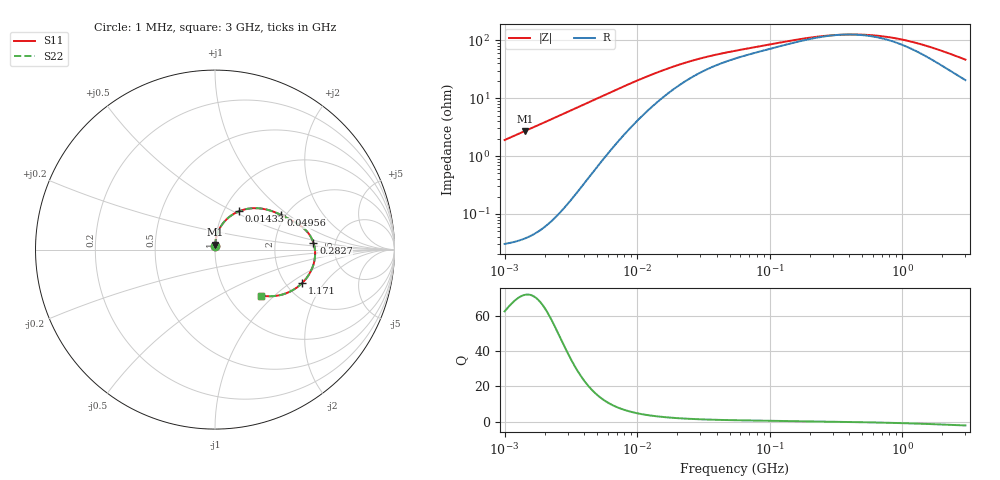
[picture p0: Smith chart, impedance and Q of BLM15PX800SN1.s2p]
! BLM15PX800SN1
# Hz S RI R 50
!Freq.(Hz) S11(Real) S11(Imag) S21(Real) S21(Imag) S12(Real) S12(Imag) S22(Real) S22(Imag)
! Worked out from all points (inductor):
!   401 points, 1 MHz to 3 GHz, reference 50 ohm
!   read as one part in series: L = 302 nH near 1.041 MHz
!   highest Q = 71.8 at 1.434 MHz (marker M1), where L = 302 nH
!   self-resonance near 369.7 MHz
!   S11 on the Smith chart (normalised r, x): 1 MHz: 1.00, +0.04; 14.33 MHz: 1.17, +0.53; 49.56 MHz: 1.90, +0.88; 282.7 MHz: 3.40, +0.37; 1.171 GHz: 2.43, -1.25; 3 GHz: 1.41, -0.83
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1000000  0.000661 0.0189  0.9993 -0.0189  0.9993 -0.0189  0.000661 0.0189
1433740  0.00112 0.0272  0.9989 -0.0272  0.9989 -0.0272  0.00112 0.0272
3823119  0.0085 0.0741  0.9915 -0.0741  0.9915 -0.0741  0.0085 0.0741
5705239  0.0218 0.1102  0.9782 -0.1102  0.9782 -0.1102  0.0218 0.1102
7858845  0.0446 0.1467  0.9554 -0.1467  0.9554 -0.1467  0.0446 0.1467
1.082539e7  0.0837 0.1852  0.9163 -0.1852  0.9163 -0.1852  0.0837 0.1852
1.432659e7  0.1325 0.2131  0.8675 -0.2131  0.8675 -0.2131  0.1325 0.2131
1.461624e7  0.1364 0.2147  0.8636 -0.2147  0.8636 -0.2147  0.1364 0.2147
1.934349e7  0.1952 0.2293  0.8048 -0.2293  0.8048 -0.2293  0.1952 0.2293
2.559965e7  0.2552 0.229  0.7448 -0.229  0.7448 -0.229  0.2552 0.229
3.456417e7  0.3126 0.2159  0.6874 -0.2159  0.6874 -0.2159  0.3126 0.2159
4.955604e7  0.3685 0.1929  0.6315 -0.1929  0.6315 -0.1929  0.3685 0.1929
5.477226e7  0.3819 0.1863  0.6181 -0.1863  0.6181 -0.1863  0.3819 0.1863
1.195584e8  0.4756 0.1337  0.5244 -0.1337  0.5244 -0.1337  0.4756 0.1337
2.094008e8  0.5303 0.0769  0.4697 -0.0769  0.4697 -0.0769  0.5303 0.0769
2.827291e8  0.5486 0.038  0.4514 -0.038  0.4514 -0.038  0.5486 0.038
4.853736e8  0.5569 -0.0412  0.4431 0.0412  0.4431 0.0412  0.5569 -0.0412
8.005644e8  0.5323 -0.1233  0.4677 0.1233  0.4677 0.1233  0.5323 -0.1233
1.171007e9  0.4848 -0.1873  0.5152 0.1873  0.5152 0.1873  0.4848 -0.1873
1.931433e9  0.3766 -0.25  0.6234 0.25  0.6234 0.25  0.3766 -0.25
2.407135e9  0.3177 -0.2598  0.6823 0.2598  0.6823 0.2598  0.3177 -0.2598
3e9  0.2586 -0.2559  0.7414 0.2559  0.7414 0.2559  0.2586 -0.2559
